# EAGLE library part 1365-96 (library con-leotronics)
DUAL ROW STRAIGHT HEADER 1364 SERIES. 1.27mm x 1.27mm. Without Fixing Post. SMT Source: http://www.leotronics.co.uk/Conexcon/Data%20Sheets/sec.%20A/1364ing.pdf
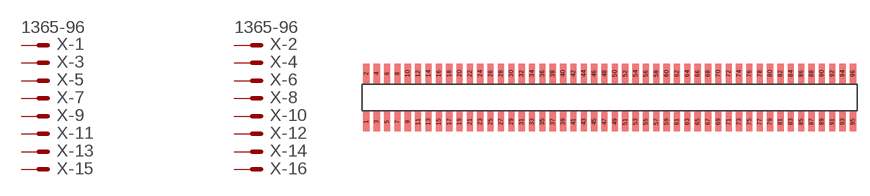
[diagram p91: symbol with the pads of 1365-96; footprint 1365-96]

Designator prefix X; gates -1=MVAL -2=MVAL -3=M -4=M -5=M -6=M -7=M -8=M -9=M -10=M -11=M -12=M -13=M -14=M -15=M -16=M -17=M -18=M -19=M -20=M -21=M -22=M -23=M -24=M -25=M -26=M -27=M -28=M -29=M -30=M -31=M -32=M -33=M -34=M -35=M -36=M -37=M -38=M -39=M -40=M -41=M -42=M -43=M -44=M -45=M -46=M -47=M -48=M -49=M -50=M -51=M -52=M -53=M -54=M -55=M -56=M -57=M -58=M -59=M -60=M -61=M -62=M -63=M -64=M -65=M -66=M -67=M -68=M -69=M -70=M -71=M -72=M -73=M -74=M -75=M -76=M -77=M -78=M -79=M -80=M -81=M -82=M -83=M -84=M -85=M -86=M -87=M -88=M -89=M -90=M -91=M -92=M -93=M -94=M -95=M -96=M

## 1365-96 (OC_FARNELL: unknown; OC_NEWARK: unknown)  [1365-96]
1  -1:S  pas
2  -2:S  pas
3  -3:S  pas
4  -4:S  pas
5  -5:S  pas
6  -6:S  pas
7  -7:S  pas
8  -8:S  pas
9  -9:S  pas
10  -10:S  pas
11  -11:S  pas
12  -12:S  pas
13  -13:S  pas
14  -14:S  pas
15  -15:S  pas
16  -16:S  pas
17  -17:S  pas
18  -18:S  pas
19  -19:S  pas
20  -20:S  pas
21  -21:S  pas
22  -22:S  pas
23  -23:S  pas
24  -24:S  pas
25  -25:S  pas
26  -26:S  pas
27  -27:S  pas
28  -28:S  pas
29  -29:S  pas
30  -30:S  pas
31  -31:S  pas
32  -32:S  pas
33  -33:S  pas
34  -34:S  pas
35  -35:S  pas
36  -36:S  pas
37  -37:S  pas
38  -38:S  pas
39  -39:S  pas
40  -40:S  pas
41  -41:S  pas
42  -42:S  pas
43  -43:S  pas
44  -44:S  pas
45  -45:S  pas
46  -46:S  pas
47  -47:S  pas
48  -48:S  pas
49  -49:S  pas
50  -50:S  pas
51  -51:S  pas
52  -52:S  pas
53  -53:S  pas
54  -54:S  pas
55  -55:S  pas
56  -56:S  pas
57  -57:S  pas
58  -58:S  pas
59  -59:S  pas
60  -60:S  pas
61  -61:S  pas
62  -62:S  pas
63  -63:S  pas
64  -64:S  pas
65  -65:S  pas
66  -66:S  pas
67  -67:S  pas
68  -68:S  pas
69  -69:S  pas
70  -70:S  pas
71  -71:S  pas
72  -72:S  pas
73  -73:S  pas
74  -74:S  pas
75  -75:S  pas
76  -76:S  pas
77  -77:S  pas
78  -78:S  pas
79  -79:S  pas
80  -80:S  pas
81  -81:S  pas
82  -82:S  pas
83  -83:S  pas
84  -84:S  pas
85  -85:S  pas
86  -86:S  pas
87  -87:S  pas
88  -88:S  pas
89  -89:S  pas
90  -90:S  pas
91  -91:S  pas
92  -92:S  pas
93  -93:S  pas
94  -94:S  pas
95  -95:S  pas
96  -96:S  pas

## Footprint 1365-96 (pad centres in mm)
DUAL ROW STRAIGHT HEADER 1364 SERIES. 1.27mm x 1.27mm. Without Fixing Post. SMT Source: http://www.leotronics.co.uk/Conexcon/Data%20Sheets/sec.%20A/1364ing.pdf
smd 0.76 x 2.4: 1 -29.845,-2.95; 2 -29.845,2.95; 3 -28.575,-2.95; 4 -28.575,2.95; 5 -27.305,-2.95; 6 -27.305,2.95; 7 -26.035,-2.95; 8 -26.035,2.95; 9 -24.765,-2.95; 10 -24.765,2.95; 11 -23.495,-2.95; 12 -23.495,2.95; 13 -22.225,-2.95; 14 -22.225,2.95; 15 -20.955,-2.95; 16 -20.955,2.95; 17 -19.685,-2.95; 18 -19.685,2.95; 19 -18.415,-2.95; 20 -18.415,2.95; 21 -17.145,-2.95; 22 -17.145,2.95; 23 -15.875,-2.95; 24 -15.875,2.95; 25 -14.605,-2.95; 26 -14.605,2.95; 27 -13.335,-2.95; 28 -13.335,2.95; 29 -12.065,-2.95; 30 -12.065,2.95; 31 -10.795,-2.95; 32 -10.795,2.95; 33 -9.525,-2.95; 34 -9.525,2.95; 35 -8.255,-2.95; 36 -8.255,2.95; 37 -6.985,-2.95; 38 -6.985,2.95; 39 -5.715,-2.95; 40 -5.715,2.95; 41 -4.445,-2.95; 42 -4.445,2.95; 43 -3.175,-2.95; 44 -3.175,2.95; 45 -1.905,-2.95; 46 -1.905,2.95; 47 -0.635,-2.95; 48 -0.635,2.95; 49 0.635,-2.95; 50 0.635,2.95; 51 1.905,-2.95; 52 1.905,2.95; 53 3.175,-2.95; 54 3.175,2.95; 55 4.445,-2.95; 56 4.445,2.95; 57 5.715,-2.95; 58 5.715,2.95; 59 6.985,-2.95; 60 6.985,2.95; 61 8.255,-2.95; 62 8.255,2.95; 63 9.525,-2.95; 64 9.525,2.95; 65 10.795,-2.95; 66 10.795,2.95; 67 12.065,-2.95; 68 12.065,2.95; 69 13.335,-2.95; 70 13.335,2.95; 71 14.605,-2.95; 72 14.605,2.95; 73 15.875,-2.95; 74 15.875,2.95; 75 17.145,-2.95; 76 17.145,2.95; 77 18.415,-2.95; 78 18.415,2.95; 79 19.685,-2.95; 80 19.685,2.95; 81 20.955,-2.95; 82 20.955,2.95; 83 22.225,-2.95; 84 22.225,2.95; 85 23.495,-2.95; 86 23.495,2.95; 87 24.765,-2.95; 88 24.765,2.95; 89 26.035,-2.95; 90 26.035,2.95; 91 27.305,-2.95; 92 27.305,2.95; 93 28.575,-2.95; 94 28.575,2.95; 95 29.845,-2.95; 96 29.845,2.95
